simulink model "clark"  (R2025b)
settings: Solver=FixedStepAuto  StartTime=0.0  StopTime=10.0  FixedStep=1e-4  RelTol=1e-3
undefined symbols (not defined in the file): DiscIntNeverNeededParam

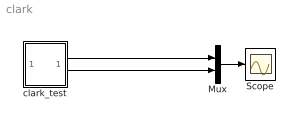
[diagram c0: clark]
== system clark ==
  Mux : Mux  Inputs=2
  Scope : Scope
  clark_test : Subsystem  TreatAsAtomicUnit=on
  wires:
  Mux/1 -> Scope/1
  clark_test/1(ialpha) -> Mux/1
  clark_test/2(ibeta) -> Mux/2

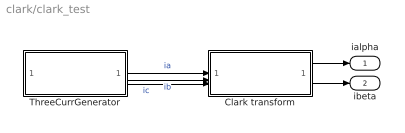
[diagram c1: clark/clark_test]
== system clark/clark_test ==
  Clark transform : Subsystem
  ThreeCurrGenerator : Subsystem
  ialpha : Outport
  ibeta : Outport  Port=2
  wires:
  Clark transform/1(ialpha) -> ialpha/1
  Clark transform/2(ibeta) -> ibeta/1
  ThreeCurrGenerator/1(ia) -> Clark transform/1(ia)  "ia"
  ThreeCurrGenerator/2(ib) -> Clark transform/2(ib)  "ib"
  ThreeCurrGenerator/3(ic) -> Clark transform/3(ic)  "ic"

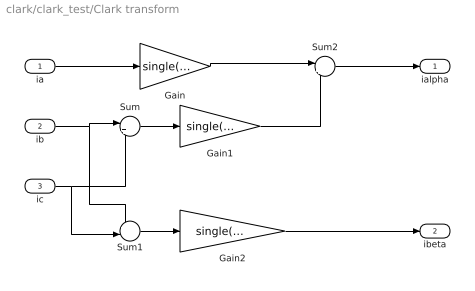
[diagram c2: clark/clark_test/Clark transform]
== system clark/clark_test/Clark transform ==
  ia : Inport
  ib : Inport  Port=2
  ic : Inport  Port=3
  Gain : Gain  Gain=single(2/3)
  Gain1 : Gain  Gain=single(1/3)
  Gain2 : Gain  Gain=single(sqrt(3)/3)
  Sum : Sum  Inputs=|++
  Sum1 : Sum  Inputs=+-|
  Sum2 : Sum  Inputs=|+-
  ialpha : Outport
  ibeta : Outport  Port=2
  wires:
  ia/1 -> Gain/1
  ib/1 -> Sum1/1, Sum/1
  ic/1 -> Sum1/2, Sum/2
  Sum/1 -> Gain1/1
  Sum1/1 -> Gain2/1
  Gain/1 -> Sum2/1
  Gain1/1 -> Sum2/2
  Gain2/1 -> ibeta/1
  Sum2/1 -> ialpha/1

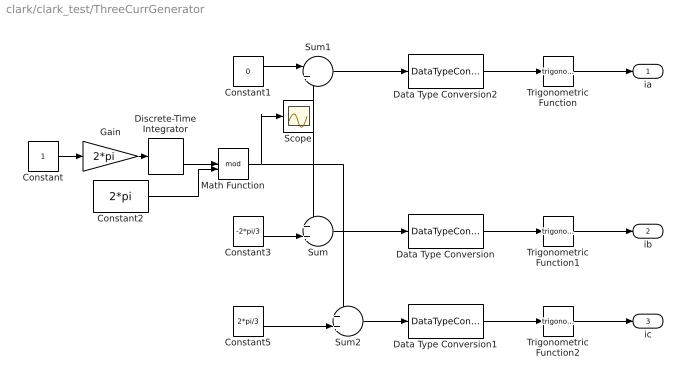
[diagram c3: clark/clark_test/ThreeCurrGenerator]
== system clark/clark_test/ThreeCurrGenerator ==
  Constant : Constant
  Constant1 : Constant  Value=0
  Constant2 : Constant  Value=2*pi
  Constant3 : Constant  Value=-2*pi/3
  Constant5 : Constant  Value=2*pi/3
  Data Type Conversion : DataTypeConversion  OutDataTypeStr=single
  Data Type Conversion1 : DataTypeConversion  OutDataTypeStr=single
  Data Type Conversion2 : DataTypeConversion  OutDataTypeStr=single
  Discrete-Time Integrator : DiscreteIntegrator  SampleTime=0.0001  ICPrevOutput=DiscIntNeverNeededParam  ICPrevScaledInput=DiscIntNeverNeededParam
  Gain : Gain  Gain=2*pi
  Math Function : Math  Operator=mod
  Scope : Scope
  Sum : Sum  Inputs=++|
  Sum1 : Sum  Inputs=|++
  Sum2 : Sum  Inputs=++|
  Trigonometric Function : Trigonometry
  Trigonometric Function1 : Trigonometry
  Trigonometric Function2 : Trigonometry
  ia : Outport
  ib : Outport  Port=2
  ic : Outport  Port=3
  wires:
  Constant/1 -> Gain/1
  Gain/1 -> Discrete-Time Integrator/1
  Constant3/1 -> Sum/2
  Constant1/1 -> Sum1/1
  Sum1/1 -> Data Type Conversion2/1
  Sum/1 -> Data Type Conversion/1
  Sum2/1 -> Data Type Conversion1/1
  Constant5/1 -> Sum2/2
  Data Type Conversion2/1 -> Trigonometric Function/1
  Trigonometric Function/1 -> ia/1
  Data Type Conversion/1 -> Trigonometric Function1/1
  Trigonometric Function1/1 -> ib/1
  Data Type Conversion1/1 -> Trigonometric Function2/1
  Trigonometric Function2/1 -> ic/1
  Discrete-Time Integrator/1 -> Math Function/1
  Constant2/1 -> Math Function/2
  Math Function/1 -> Sum2/1, Sum1/2, Sum/1, Scope/1
